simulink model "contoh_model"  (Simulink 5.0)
settings: Solver=ode45  StartTime=0.0  StopTime=40.0  RelTol=1e-6

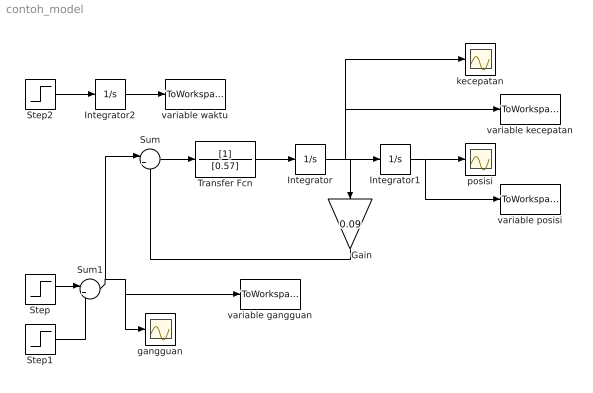
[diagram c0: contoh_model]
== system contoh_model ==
  Gain : Gain  Orientation=down  Gain=0.09
  Integrator : Integrator
  Integrator1 : Integrator
  Integrator2 : Integrator
  Step : Step  Time=0.5  SampleTime=0
  Step1 : Step  Time=1.5  SampleTime=0
  Step2 : Step  Time=0  SampleTime=0
  Sum : Sum  Inputs=|+-
  Sum1 : Sum  Inputs=|+-
  Transfer Fcn : TransferFcn  Denominator=[0.57]
  gangguan : Scope
  kecepatan : Scope
  posisi : Scope
  variable gangguan : ToWorkspace  VariableName=gangguan  SampleTime=-1  SaveFormat=Array
  variable kecepatan : ToWorkspace  VariableName=kecepatan  SampleTime=-1  SaveFormat=Array
  variable posisi : ToWorkspace  VariableName=posisi  SampleTime=-1  SaveFormat=Array
  variable waktu : ToWorkspace  VariableName=time  SampleTime=-1  SaveFormat=Array
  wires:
  Integrator/1 -> Integrator1/1, Gain/1, kecepatan/1, variable kecepatan/1
  Integrator1/1 -> posisi/1, variable posisi/1
  Transfer Fcn/1 -> Integrator/1
  Sum/1 -> Transfer Fcn/1
  Step/1 -> Sum1/1
  Step1/1 -> Sum1/2
  Sum1/1 -> Sum/1, gangguan/1, variable gangguan/1
  Gain/1 -> Sum/2
  Step2/1 -> Integrator2/1
  Integrator2/1 -> variable waktu/1
